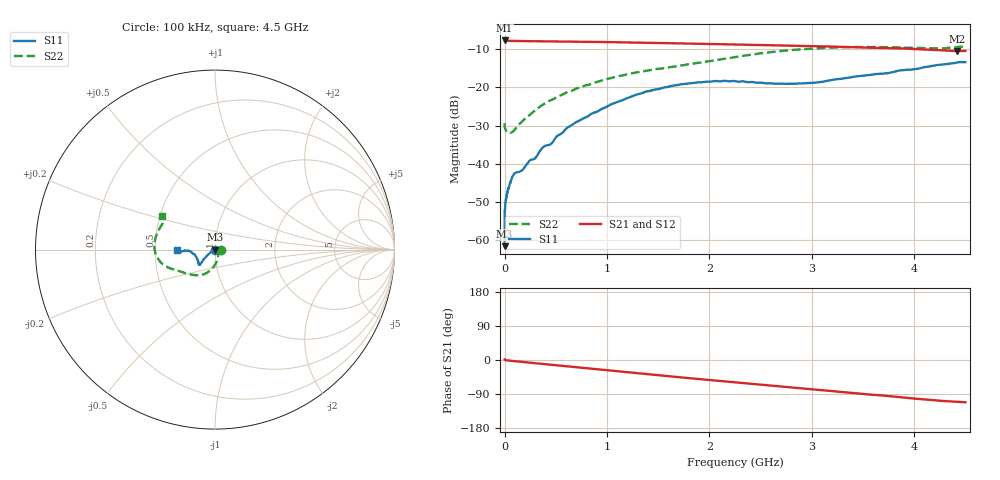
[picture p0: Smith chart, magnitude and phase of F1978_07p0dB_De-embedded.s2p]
! Integrated Device Technology
! Corporate Headquarters
! 6024 Silver Creek Valley Road
! San Jose, CA 95138  USA
! Phone:  1-408-284-8200
! Toll Free:  1-800-223-1366
! Webpage:  http://www.idt.com/
! Timing and RF Division
! 515 Groton Road, Suite 102
! Westford, MA 01886-6024
! Device:  F1978
! Description: 6-bit, 75 ohm, 0.5 dB Digital Step Attenuator
! Frequency:  5.0 MHz -  3.00 GHz
! Package:  4x4 mm QFN Plastic Package: 20 pin
! Ports:  2 RF, 11 DC
!  Pin  1  = D5 (16 dB)
!  Pin  2  = RF1  =  Port 1
!  Pin  3  = Serial Data In (DATA)
!  Pin  4  = Serial Clock (CLK)
!  Pin  5  = Serial Latch Enable (LE)
!  Pin  6  = VDD
!  Pin  7  = NC
!  Pin  8  = NC
!  Pin  9  = NC
!  Pin 10  = GND
!  Pin 11  = GND
!  Pin 12  = NC
!  Pin 13  = VMODE
!  Pin 14  = RF2  =  Port 2
!  Pin 15  = D4 (8 dB)
!  Pin 16  = D3 (4 dB)
!  Pin 17  = D2 (2 dB)
!  Pin 18  = NC
!  Pin 19  = D1 (1 dB)
!  Pin 20  = D0 (0.5 dB)
! State:  14
! Atten State:  7.0 dB
! Voltage:  +3.30 Volts
! Current:  0.594 mA
! Data:  The device was measured on a F1975 evaluation board which has
!  individual transmission lines to the RF pins.  Data was collected
!  using a calibrated network analyzer.  The evaluation board was
!  de-embedded using Automatic Fixture Removal (AFR).
!  The reference plane is the edge of the package pin.
! Misc:
!  Action Tracker AT0416
! Date Measured:  2018-02-08
! Date:  2018-03-26  MJV
! Note:
!  Integrated Device Technology supplies this data as a sample of measured
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# GHz S dB R 75
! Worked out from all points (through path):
!   291 points, 100 kHz to 4.5 GHz, reference 75 ohm
!   highest |S21| = -7.68 dB at 100 kHz (marker M1); lowest = -10.4 dB at 4.42 GHz (marker M2)
!   group delay of S21, straight-line fit = 70.3 ps
!   lowest |S11| = -61.6 dB at 100 kHz (marker M3), VSWR 1.00, Z = 74.9 + j0.000813 ohm
!   |S11| at or under -10 dB: start of sweep to end of sweep
!   |S22| runs from -31.9 to -9.2 dB; largest |S21 - S12| = 0.00021
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0.0001  -61.64 179.6  -7.68 1.2  -7.68 1.2  -29.39 0.0
0.0004  -56.10 -167.1  -7.70 1.1  -7.70 1.1  -29.86 -2.1
0.0005  -55.12 -160.9  -7.70 1.1  -7.70 1.1  -29.94 -2.1
0.0007  -54.81 -167.7  -7.71 1.0  -7.71 1.0  -30.11 -2.6
0.0008  -53.60 -162.4  -7.71 1.0  -7.71 1.0  -30.16 -2.2
0.002  -52.10 -164.9  -7.73 0.8  -7.73 0.8  -30.56 -2.9
0.011  -49.45 -158.4  -7.76 -0.5  -7.75 -0.5  -31.18 -9.6
0.036  -46.45 -160.7  -7.78 -1.3  -7.78 -1.3  -31.71 -19.8
0.08  -43.18 -149.5  -7.81 -2.5  -7.81 -2.5  -31.64 -37.5
0.3  -38.55 -145.2  -7.89 -8.5  -7.89 -8.5  -25.98 -73.2
0.36  -36.12 -147.1  -7.91 -10.1  -7.91 -10.1  -24.76 -77.0
0.46  -34.69 -148.0  -7.94 -12.8  -7.93 -12.8  -23.26 -83.0
0.62  -30.44 -147.7  -7.99 -17.0  -7.98 -17.0  -21.18 -90.8
0.76  -28.25 -145.1  -8.03 -20.8  -8.02 -20.8  -19.77 -97.2
1.04  -24.43 -142.4  -8.12 -28.2  -8.12 -28.2  -17.52 -108.0
1.52  -20.33 -136.9  -8.34 -40.7  -8.34 -40.7  -15.08 -126.0
1.88  -18.70 -135.2  -8.55 -49.8  -8.55 -49.8  -13.58 -140.6
2.26  -18.39 -138.5  -8.75 -59.2  -8.74 -59.2  -12.01 -153.3
3.02  -18.80 -165.1  -9.19 -77.8  -9.18 -77.8  -9.80 -171.9
3.76  -16.17 -177.5  -9.68 -95.4  -9.68 -95.4  -9.47 166.1
4.42  -13.45 -177.0  -10.45 -110.3  -10.44 -110.3  -9.40 149.2
4.5  -13.37 -179.1  -10.42 -111.6  -10.42 -111.6  -9.16 147.8
